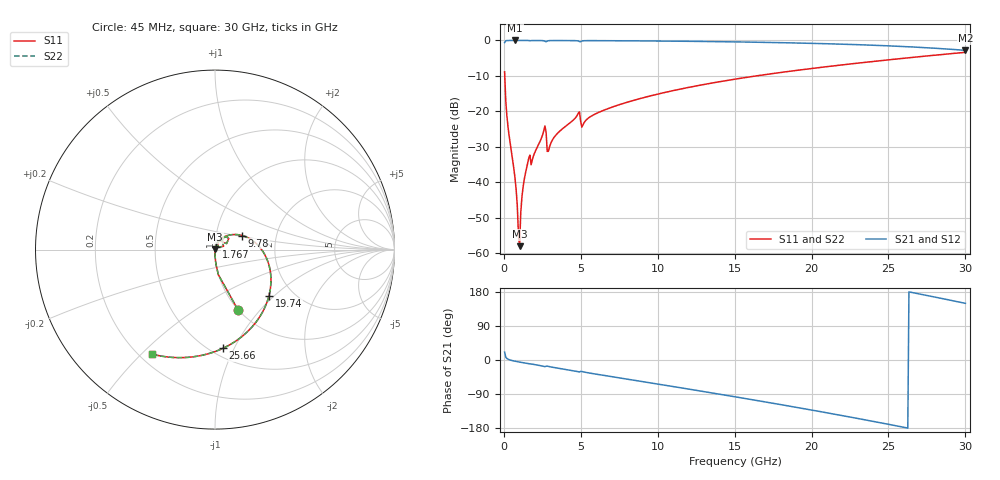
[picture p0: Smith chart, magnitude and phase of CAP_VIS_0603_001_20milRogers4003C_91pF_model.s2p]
! S-parameter model data by Modelithics Inc.  support@modelithics.com  813-866-6335  Tampa FL USA
! S-Parameter data specifications:
! Substrate: 20-mil Rogers 4003C, substrate thickness, H=0.508mm, Dielectric constant, Er=3.75
! PCB Mounting Pad Footprint: Pad width, PadW=0.90mm , Pad length, PadL=1.00mm , Pad gap, PadG (edge-to-edge)=1.00mm , Reference planes=3.0mm apart
! Created Wed Nov 18 13:30:52 2015
# hz S ma R 50
! 2 Port Network Data from SP1.SP block
! freq  magS11  angS11  magS21  angS21  magS12  angS12  magS22  angS22
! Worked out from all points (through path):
!   401 points, 45 MHz to 30 GHz, reference 50 ohm
!   highest |S21| = -0.01 dB at 719 MHz (marker M1); lowest = -2.8 dB at 30 GHz (marker M2)
!   group delay of S21, straight-line fit = 19.4 ps
!   lowest |S11| = -58.0 dB at 1.019 GHz (marker M3), VSWR 1.00, Z = 50.1 + j0.0947 ohm
!   |S11| at or under -10 dB: 55.49 MHz to 16.39 GHz (16.33 GHz wide, 199 % of centre)
!   |S22| runs from -58.0 to -3.4 dB; largest |S21 - S12| = 0
!   S11 on the Smith chart (normalised r, x): 45 MHz: 1.00, -0.77; 1.767 GHz: 1.02, +0.03; 9.78 GHz: 1.34, +0.22; 19.74 GHz: 1.52, -0.93; 25.66 GHz: 0.57, -0.91; 30 GHz: 0.25, -0.54
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4.5e7  0.3604 -69.1  0.9326 20.9  0.9326 20.9  0.3604 -69.1
2.696625e8  0.05978 -87.6  0.9978 2.0  0.9978 2.0  0.05978 -87.6
7.189875e8  0.0116 -90.1  0.9992 -3.2  0.9992 -3.2  0.0116 -90.1
8.687625e8  0.004745 -86.1  0.9992 -4.4  0.9992 -4.4  0.004745 -86.1
1.018538e9  0.001265 48.3  0.9992 -5.5  0.9992 -5.5  0.001265 48.3
1.093425e9  0.003693 71.8  0.9991 -6.1  0.9991 -6.1  0.003693 71.8
1.2432e9  0.008515 77.1  0.999 -7.1  0.999 -7.1  0.008515 77.1
1.392975e9  0.01323 77.5  0.9988 -8.2  0.9988 -8.2  0.01323 77.5
1.54275e9  0.01852 75.9  0.9982 -9.3  0.9982 -9.3  0.01852 75.9
1.767412e9  0.01773 64.1  0.995 -10.4  0.995 -10.4  0.01773 64.1
2.591175e9  0.0535 63.1  0.989 -16.9  0.989 -16.9  0.0535 63.1
2.965612e9  0.03165 62.3  0.9937 -17.6  0.9937 -17.6  0.03165 62.3
4.762912e9  0.08807 54.8  0.9885 -30.5  0.9885 -30.5  0.08807 54.8
5.062462e9  0.06004 42.4  0.9801 -30.3  0.9801 -30.3  0.06004 42.4
9.780375e9  0.1709 27.2  0.9822 -62.0  0.9822 -62.0  0.1709 27.2
1.007992e10  0.1771 25.3  0.981 -64.0  0.981 -64.0  0.1771 25.3
1.50225e10  0.2848 -7.6  0.9544 -97.0  0.9544 -97.0  0.2848 -7.6
1.974041e10  0.396 -40.6  0.9129 -130.2  0.9129 -130.2  0.396 -40.6
2.003996e10  0.4034 -42.8  0.9096 -132.3  0.9096 -132.3  0.4034 -42.8
2.505742e10  0.5346 -80.6  0.8381 -170.1  0.8381 -170.1  0.5346 -80.6
2.565652e10  0.5514 -85.3  0.827 -174.9  0.827 -174.9  0.5514 -85.3
3e10  0.6794 -120.9  0.7246 149.5  0.7246 149.5  0.6794 -120.9
